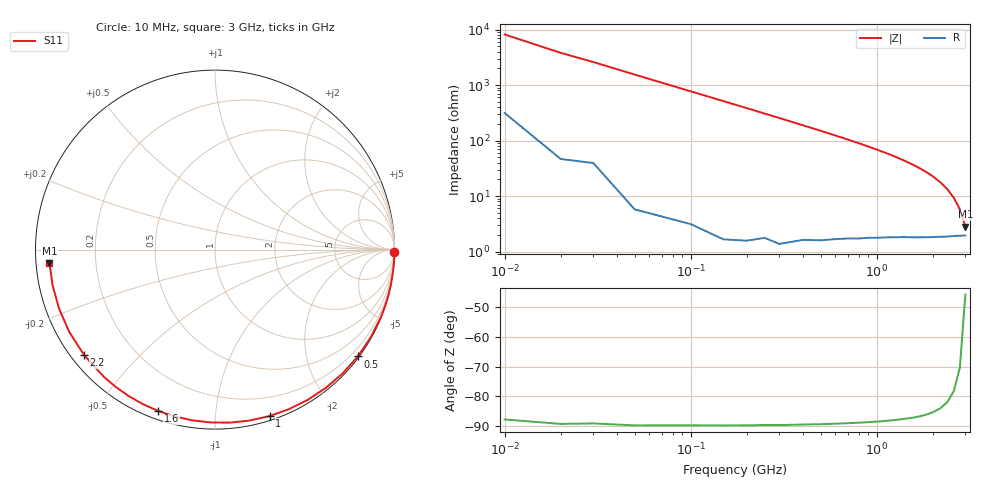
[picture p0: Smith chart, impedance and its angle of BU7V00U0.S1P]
! SIEMENS Small Signal Semiconductors
! BB833
! Si Tuning Diode in SOD323
! VR = 7 V
! S-Parameters:  April  1996
# GHz  S  MA  R  50
!  f  S11
! GHz  MAG  ANG
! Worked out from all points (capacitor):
!   31 points, 10 MHz to 3 GHz, reference 50 ohm
!   read as one part to ground: C = 2.04 pF near 10 MHz
!   lowest |Z| = 2.8 ohm at 3 GHz (marker M1)
!   S11 on the Smith chart (normalised r, x): 10 MHz: open; 500 MHz: 0.03, -3.01; 1 GHz: 0.04, -1.38; 1.6 GHz: 0.04, -0.71; 2.2 GHz: 0.04, -0.35; 3 GHz: 0.04, -0.04
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0.01  0.9995 -0.7
0.05  0.9998 -3.7
0.1  0.9995 -7.4
0.15  0.9994 -11.1
0.2  0.999 -14.8
0.3  0.998 -22.2
0.4  0.9958 -29.6
0.5  0.9937 -36.8
0.6  0.9906 -44.1
0.7  0.9872 -51.2
0.8  0.9839 -58.2
0.9  0.9797 -65.1
1  0.976 -71.8
1.1  0.9717 -78.5
1.2  0.9677 -84.9
1.3  0.9636 -91.3
1.4  0.9597 -97.5
1.5  0.9562 -103.5
1.6  0.9533 -109.3
1.7  0.9501 -115.0
1.8  0.9468 -120.6
1.9  0.9441 -125.9
2  0.9413 -131.1
2.2  0.9366 -141.1
2.4  0.9327 -150.5
2.6  0.929 -159.3
2.8  0.9266 -167.6
3  0.9251 -175.4
